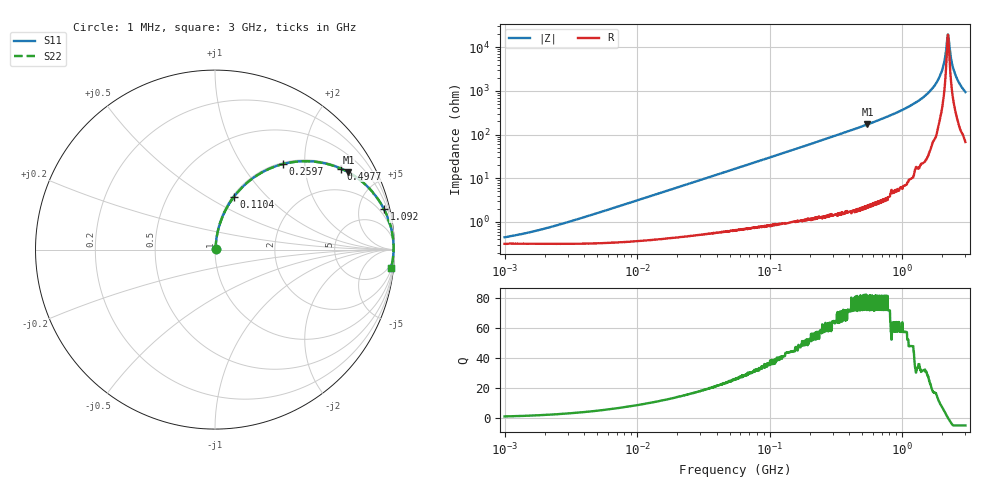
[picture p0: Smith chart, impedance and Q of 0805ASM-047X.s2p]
!s-Parameter Generated by FASTRON Sdn. Bhd.
!FASTRON P/N : 0805ASM-047X
!Keysight Technologies: E4991B_MY54100416_A.01.15
!Date: Fri Jun 19 14:49:07 2026
!Version  :Rev00  Fri Jun 19 14:49:07 2026
!Data & Calibration Information:
!Freq  S11  S21  S12  S22
!PortZ  Port1:50+j0  Port2:50+j0
!When reading reference impedance value at option line is always used.
! Remarks : This data is being provided solely for informational purposes.
# Hz S dB R 50
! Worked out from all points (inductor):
!   1601 points, 1 MHz to 3 GHz, reference 50 ohm
!   read as one part in series: L = 49.9 nH near 3.037 MHz
!   highest Q = 81.5 at 547.3 MHz (marker M1), where L = 49.8 nH
!   self-resonance near 2.211 GHz
!   S11 on the Smith chart (normalised r, x): 1 MHz: 1.01, +0.01; 110.4 MHz: 1.02, +0.66; 259.7 MHz: 1.03, +1.56; 497.7 MHz: 1.04, +3.09; 1.092 GHz: 1.15, +8.36; 3 GHz: 2, -19
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1000000  -47.00 44.8  -0.03 -0.2  -0.03 -0.2  -47.00 44.8
3804036  -38.20 74.4  -0.03 -0.7  -0.03 -0.7  -38.20 74.4
1.447069e7  -27.00 82.3  -0.04 -2.5  -0.04 -2.5  -27.00 82.3
5.504702e7  -15.80 78.4  -0.17 -9.4  -0.17 -9.4  -15.80 78.4
1.103592e8  -10.10 70.4  -0.52 -18.1  -0.52 -18.1  -10.10 70.4
2.083556e8  -5.60 57.3  -1.50 -31.6  -1.50 -31.6  -5.60 57.3
2.596726e8  -4.30 51.5  -2.13 -37.6  -2.13 -37.6  -4.30 51.5
4.976708e8  -1.57 32.7  -5.34 -56.5  -5.34 -56.5  -1.57 32.7
5.473095e8  -1.32 30.1  -6.00 -59.2  -6.00 -59.2  -1.32 30.1
7.925923e8  -0.61 20.5  -9.13 -68.7  -9.13 -68.7  -0.61 20.5
1.091779e9  -0.28 13.4  -12.70 -75.5  -12.70 -75.5  -0.28 13.4
1.466741e9  -0.11 7.6  -17.60 -80.6  -17.60 -80.6  -0.11 7.6
1.791767e9  -0.06 3.9  -23.30 -82.6  -23.30 -82.6  -0.06 3.9
2.000286e9  -0.04 1.9  -29.40 -80.3  -29.40 -80.3  -0.04 1.9
2.071593e9  -0.04 1.3  -32.90 -77.0  -32.90 -77.0  -0.04 1.3
2.156205e9  -0.04 0.5  -39.80 -61.7  -39.80 -61.7  -0.04 0.5
2.210833e9  -0.04 0.1  -45.90 -10.5  -45.90 -10.5  -0.04 0.1
2.266846e9  -0.05 -0.4  -41.00 54.0  -41.00 54.0  -0.05 -0.4
2.39512e9  -0.05 -1.4  -31.70 76.0  -31.70 76.0  -0.05 -1.4
2.51802e9  -0.06 -2.4  -27.50 79.1  -27.50 79.1  -0.06 -2.4
2.727913e9  -0.08 -4.0  -23.10 80.4  -23.10 80.4  -0.08 -4.0
3e9  -0.11 -6.0  -19.60 79.9  -19.60 79.9  -0.11 -6.0
